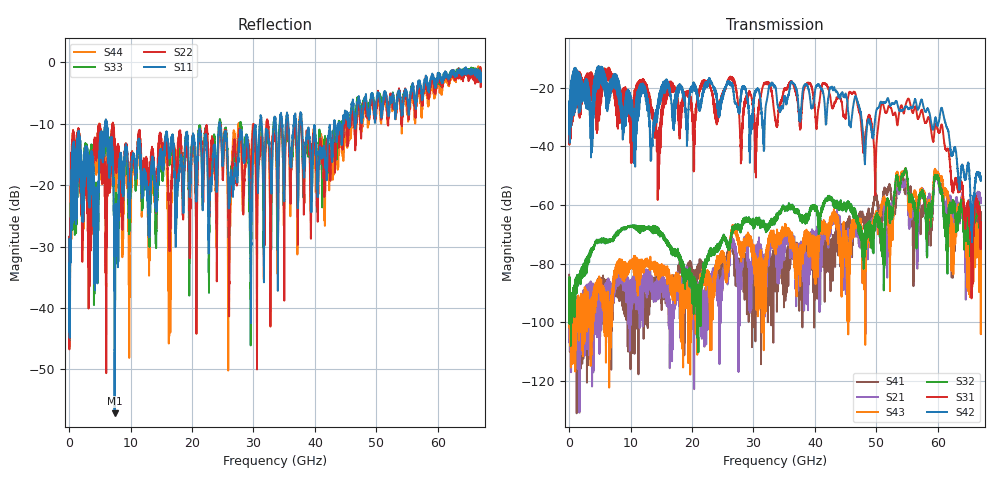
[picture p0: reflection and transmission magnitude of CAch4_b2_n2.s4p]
!Agilent Technologies,N5247A,US51170199,A.09.90.13
!Agilent N5247A: A.09.90.13
!Date: Thursday, October 18, 2018 09:31:25
!Correction: S11(Full 4 Port(1,2,3,4))
!S12(Full 4 Port(1,2,3,4))
!S13(Full 4 Port(1,2,3,4))
!S14(Full 4 Port(1,2,3,4))
!S21(Full 4 Port(1,2,3,4))
!S22(Full 4 Port(1,2,3,4))
!S23(Full 4 Port(1,2,3,4))
!S24(Full 4 Port(1,2,3,4))
!S31(Full 4 Port(1,2,3,4))
!S32(Full 4 Port(1,2,3,4))
!S33(Full 4 Port(1,2,3,4))
!S34(Full 4 Port(1,2,3,4))
!S41(Full 4 Port(1,2,3,4))
!S42(Full 4 Port(1,2,3,4))
!S43(Full 4 Port(1,2,3,4))
!S44(Full 4 Port(1,2,3,4))
!S4P File: Measurements: <S11,S12,S13,S14>,
!<S21,S22,S23,S24>,
!<S31,S32,S33,S34>,
!<S41,S42,S43,S44>:
# Hz S  dB  R 50
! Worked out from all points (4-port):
!   6701 points, 10 MHz to 67 GHz, reference 50 ohm
!   strongest paths, dB at 10 MHz, 16.76 GHz, 33.51 GHz, 50.25 GHz, 67 GHz:
!     S42: -30.5, -26.4, -19.7, -27.0, -51.6
!     S31: -30.6, -21.4, -30.5, -34.0, -73.1
!     S32: -87.4, -74.5, -64.5, -64.9, -73.0
!     S43: -88.1, -86.4, -72.5, -68.5, -67.0
!     S21: -87.9, -113.3, -76.0, -65.3, -58.2
!     S41: -83.8, -86.1, -77.5, -60.7, -63.9
!   lowest |S11| = -57.1 dB at 7.409 GHz (marker M1), VSWR 1.00, Z = 50.1 + j0.0155 ohm
!   |S11| at or under -10 dB: start of sweep to 5.859 GHz; 6.126 GHz to 24.47 GHz (18.34 GHz wide, 120 % of centre); 24.55 GHz to 31.03 GHz (6.485 GHz wide, 23.3 % of centre)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
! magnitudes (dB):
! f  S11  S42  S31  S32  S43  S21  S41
! 10 MHz  -28.8  -30.5  -30.6  -87.4  -88.1  -87.9  -83.8
! 7.409 GHz  -57.1  -16.3  -23.9  -70.3  -85.2  -86.9  -84.2
! 13.46 GHz  -17.6  -38.9  -29.6  -68.0  -80.5  -87.2  -90.4
! 41.55 GHz  -14.9  -24.9  -18.5  -59.5  -67.0  -67.1  -75.4
! 49.79 GHz  -9.5  -30.8  -54.8  -65.1  -64.9  -65.1  -57.4
! 55.18 GHz  -6.8  -27.3  -23.7  -54.3  -58.2  -60.5  -54.9
! 67 GHz  -3.2  -51.6  -73.1  -73.0  -67.0  -58.2  -63.9
